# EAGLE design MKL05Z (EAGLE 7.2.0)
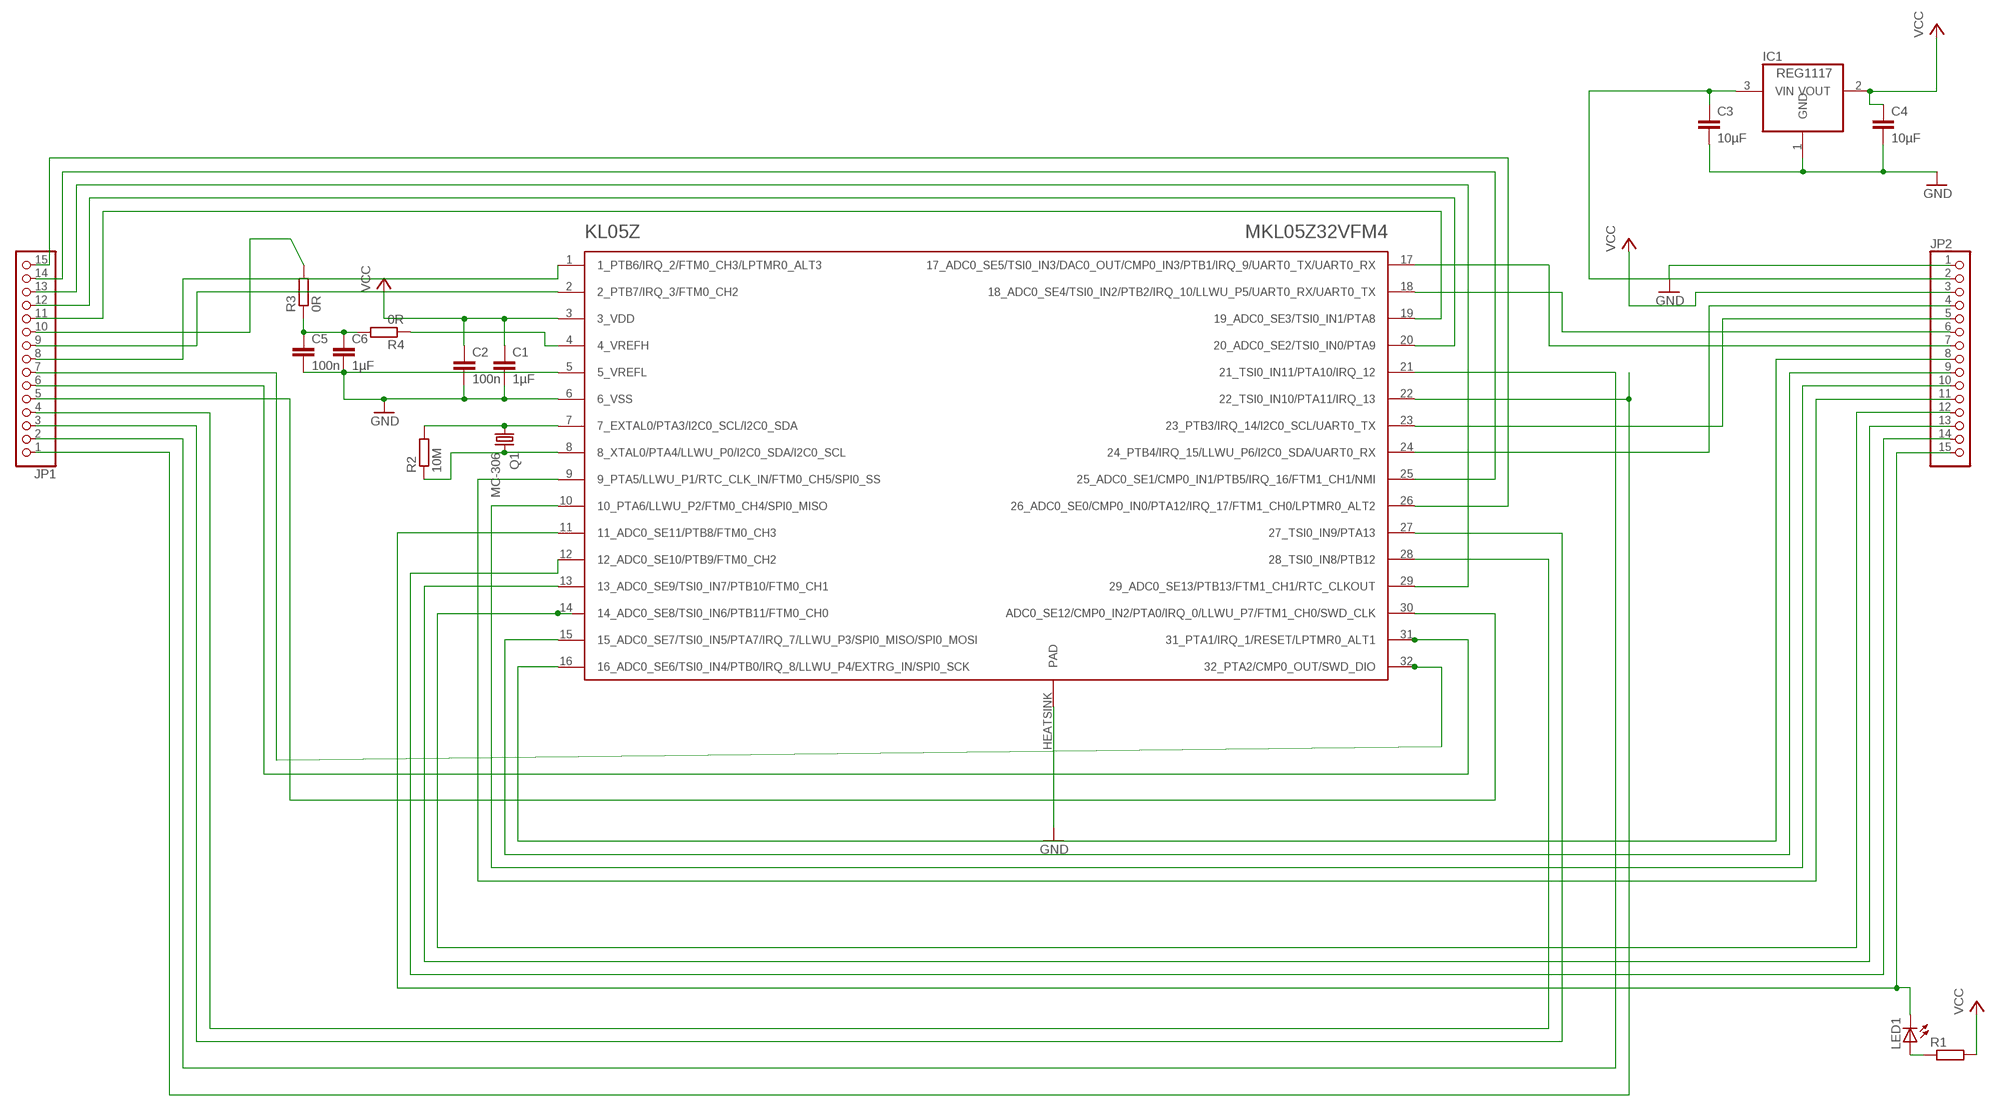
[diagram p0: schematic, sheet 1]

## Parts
C1  1µF  C-EUC0603  [C0603]
C2  100n  C-EUC0603  [C0603]
C3  10µF  C-EUC0805  [C0805]
C4  10µF  C-EUC0805  [C0805]
C5  100n  C-EUC0603  [C0603]
C6  1µF  C-EUC0603  [C0603]
IC1  REG1117  [SOT223]
JP1  PINHD-1X15  [1X15]
JP2  PINHD-1X15  [1X15]
KL05Z  MKL05Z32VFM4  MKL15Z128VFM4  [QFN32]
LED1  LEDCHIPLED_0805  [CHIPLED_0805]
Q1  MC-306  [MC-306]
R1  R-EU_R0603  [R0603]
R2  10M  R-EU_R0603  [R0603]
R3  0R  R-EU_R0402  [R0402]
R4  0R  R-EU_R0402  [R0402]

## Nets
GND: C1.2 C2.2 C3.2 C4.2 C5.2 C6.2 IC1.1(GND) JP2.1 KL05Z.5(5_VREFL) KL05Z.6(6_VSS) KL05Z.HEATSINK(PAD)
N$1: JP1.6 KL05Z.31(31_PTA1/IRQ_1/RESET/LPTMR0_ALT1)
N$2: JP1.4 KL05Z.28(28_TSI0_IN8/PTB12)
N$3: JP1.5 KL05Z.30(ADC0_SE12/CMP0_IN2/PTA0/IRQ_0/LLWU_P7/FTM1_CH0/SWD_CLK)
N$4: KL05Z.7(7_EXTAL0/PTA3/I2C0_SCL/I2C0_SDA) Q1.1 R2.2
N$6: C3.1 IC1.3(VIN) JP2.2
N$7: JP2.6 KL05Z.18(18_ADC0_SE4/TSI0_IN2/PTB2/IRQ_10/LLWU_P5/UART0_RX/UART0_TX)
N$8: JP2.7 KL05Z.17(17_ADC0_SE5/TSI0_IN3/DAC0_OUT/CMP0_IN3/PTB1/IRQ_9/UART0_TX/UART0_RX)
N$9: JP2.4 KL05Z.24(24_PTB4/IRQ_15/LLWU_P6/I2C0_SDA/UART0_RX)
N$10: JP2.5 KL05Z.23(23_PTB3/IRQ_14/I2C0_SCL/UART0_TX)
N$11: KL05Z.8(8_XTAL0/PTA4/LLWU_P0/I2C0_SDA/I2C0_SCL) Q1.4 R2.1
N$12: C5.1 C6.1 R3.1 R4.2
N$13: KL05Z.4(4_VREFH) R4.1
N$14: JP2.11 KL05Z.9(9_PTA5/LLWU_P1/RTC_CLK_IN/FTM0_CH5/SPI0_SS)
N$15: JP2.10 KL05Z.10(10_PTA6/LLWU_P2/FTM0_CH4/SPI0_MISO)
N$16: JP2.9 KL05Z.15(15_ADC0_SE7/TSI0_IN5/PTA7/IRQ_7/LLWU_P3/SPI0_MISO/SPI0_MOSI)
N$17: JP2.8 KL05Z.16(16_ADC0_SE6/TSI0_IN4/PTB0/IRQ_8/LLWU_P4/EXTRG_IN/SPI0_SCK)
N$18: JP1.7 KL05Z.32(32_PTA2/CMP0_OUT/SWD_DIO)
N$19: JP1.3 KL05Z.27(27_TSI0_IN9/PTA13)
N$20: JP1.2 KL05Z.21(21_TSI0_IN11/PTA10/IRQ_12)
N$21: JP1.1 KL05Z.22(22_TSI0_IN10/PTA11/IRQ_13)
N$22: JP1.10 R3.2
N$23: JP1.11 KL05Z.19(19_ADC0_SE3/TSI0_IN1/PTA8)
N$24: JP1.12 KL05Z.20(20_ADC0_SE2/TSI0_IN0/PTA9)
N$25: JP1.13 KL05Z.29(29_ADC0_SE13/PTB13/FTM1_CH1/RTC_CLKOUT)
N$26: JP1.15 KL05Z.26(26_ADC0_SE0/CMP0_IN0/PTA12/IRQ_17/FTM1_CH0/LPTMR0_ALT2)
N$27: JP1.14 KL05Z.25(25_ADC0_SE1/CMP0_IN1/PTB5/IRQ_16/FTM1_CH1/NMI)
N$28: LED1.A R1.1
N$29: JP1.9 KL05Z.2(2_PTB7/IRQ_3/FTM0_CH2)
N$30: JP2.12 KL05Z.14(14_ADC0_SE8/TSI0_IN6/PTB11/FTM0_CH0)
N$31: JP1.8 KL05Z.1(1_PTB6/IRQ_2/FTM0_CH3/LPTMR0_ALT3)
N$32: JP2.13 KL05Z.13(13_ADC0_SE9/TSI0_IN7/PTB10/FTM0_CH1)
N$33: JP2.14 KL05Z.12(12_ADC0_SE10/PTB9/FTM0_CH2)
N$34: JP2.15 KL05Z.11(11_ADC0_SE11/PTB8/FTM0_CH3) LED1.C
VCC: C1.1 C2.1 C4.1 IC1.2(VOUT) JP2.3 KL05Z.3(3_VDD) R1.2

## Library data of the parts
C1-C6 = rcl:C-EU: CAPACITOR, European symbol
IC1 = burr-brown:REG1117: 800mA and 1A Low Dropout (LDO) Positive Regulator 1.8V, 2.5V, 2.85V, 3.3V, 5V, and Adj; MPN: REG1117; OC_FARNELL: 1097566; OC_NEWARK: 14P6981
JP1 JP2 = pinhead:PINHD-1X15: PIN HEADER
KL05Z = kl05z32vfm4:MKL15Z128VFM4
LED1 = led:LED: LED
Q1 = crystal:MC-306: kHz RANGE CRYSTAL UNIT SMD; MPN: MC-306 60.0KHZ 100PPM ,12.5PF; OC_FARNELL: 1278040; OC_NEWARK: 31M5576
R1-R4 = rcl:R-EU_: RESISTOR, European symbol

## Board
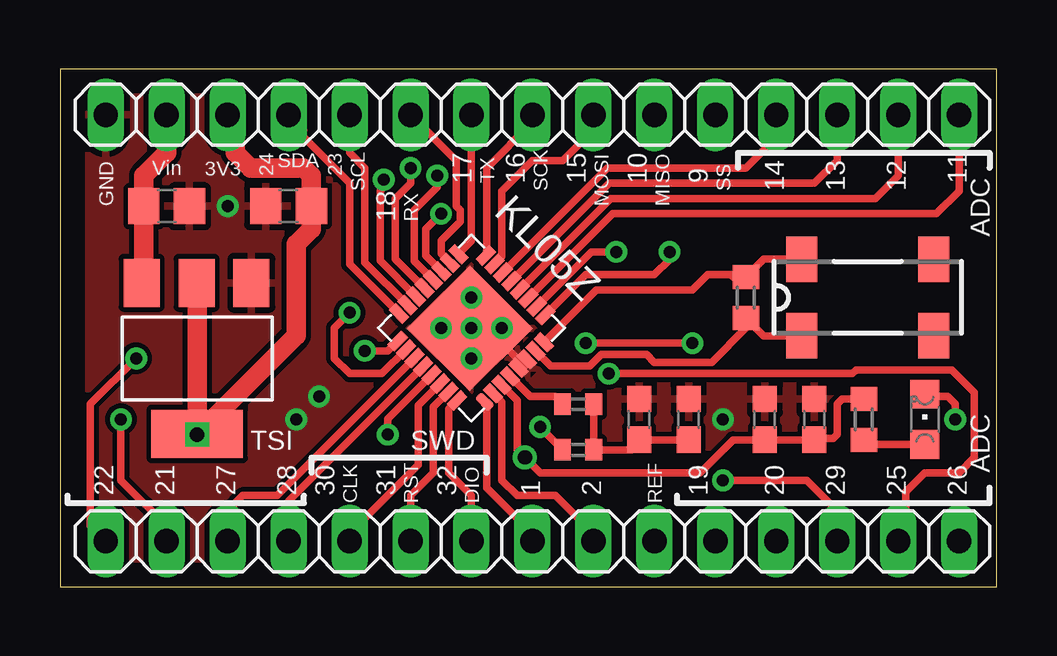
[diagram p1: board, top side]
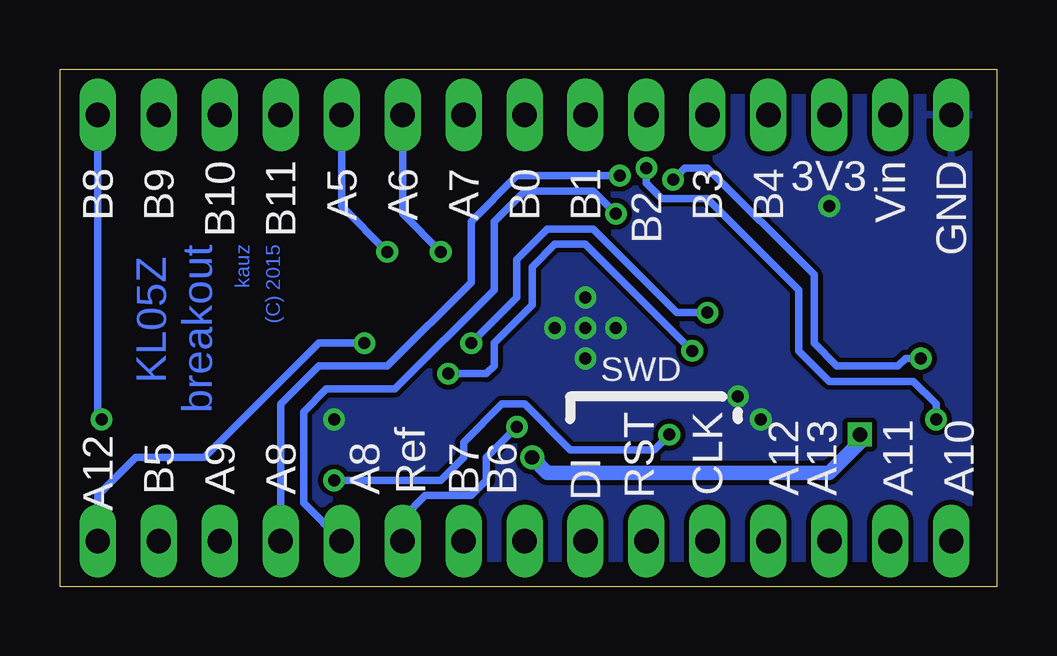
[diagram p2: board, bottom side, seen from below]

Size 39.04 x 21.58 mm. Coordinates in mm from the lower left corner, seen from the top.
Outline: 0,0 39.04,0 39.04,21.58 0,21.58 0,0
Copper layers (1*16): Top 0.035mm / dielectric 1.5mm / Bottom 0.035mm
Design rules "default *": minimum track width 10mil, minimum drill 24mil, track to track 8mil, track to pad 8mil, pad to pad 8mil, via to via 8mil, smd to smd 8mil, copper to edge 40mil, drill to drill 8mil, minimum pad ring 10mil, minimum via ring 8mil, stop-mask expansion 4mil, vias tented up to drill 0.50038125mm, thermal gap 10mil

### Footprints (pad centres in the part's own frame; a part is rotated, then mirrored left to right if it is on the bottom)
C0603 = smd 1.1 x 1: 1 -0.85,0; 2 0.85,0
C0805 = smd 1.3 x 1.5: 1 -0.95,0; 2 0.95,0
SOT223 = smd 1.499 x 2.007: 1 -2.261,-3.15; 2 0.025,-3.15; 3 2.311,-3.15 | smd 3.81 x 2.007: 4 0,3.15
1X15 = drill 1.016 long: 1 -17.78,0; 2 -15.24,0; 3 -12.7,0; 4 -10.16,0; 5 -7.62,0; 6 -5.08,0; 7 -2.54,0; 8 0,0; 9 2.54,0; 10 5.08,0; 11 7.62,0; 12 10.16,0; 13 12.7,0; 14 15.24,0; 15 17.78,0
QFN32 = smd 0.813 x 0.406: 1 -2.56,1.79; 2 -2.56,1.29; 3 -2.56,0.79; 4 -2.56,0.29; 5 -2.56,-0.21; 6 -2.56,-0.71; 7 -2.56,-1.21; 8 -2.56,-1.71; 17 2.56,-1.79; 18 2.56,-1.29; 19 2.56,-0.79; 20 2.56,-0.29; 21 2.56,0.21; 22 2.56,0.71; 23 2.56,1.21; 24 2.56,1.71 | smd 0.406 x 0.813: 9 -1.79,-2.56; 10 -1.29,-2.56; 11 -0.79,-2.56; 12 -0.29,-2.56; 13 0.21,-2.56; 14 0.71,-2.56; 15 1.21,-2.56; 16 1.71,-2.56; 25 1.79,2.56; 26 1.29,2.56; 27 0.79,2.56; 28 0.29,2.56; 29 -0.21,2.56; 30 -0.71,2.56; 31 -1.21,2.56; 32 -1.71,2.56 | smd 3.7 x 3.7: HEATSINK 0.04,0.06
CHIPLED_0805 = smd 1.2 x 1.2: A 0,-1.05; C 0,1.05
MC-306 = smd 1.3 x 1.9: 1 -2.75,-1.6; 2 2.75,-1.6; 3 2.75,1.6; 4 -2.75,1.6
R0603 = smd 1 x 1.1: 1 -0.85,0; 2 0.85,0
R0402 = smd 0.7 x 0.9: 1 -0.65,0; 2 0.65,0

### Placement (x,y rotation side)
C1  29.37,6.99 90 top
C2  31.43,6.99 90 top
C3  4.45,15.88 0 top
C4  9.53,15.88 180 top
C5  26.19,6.99 90 top
C6  24.13,6.99 90 top
IC1  5.71,9.53 180 top
JP1  19.68,1.91 0 top
JP2  19.68,19.68 0 top
KL05Z  17.14,10.79 135 top
LED1  36.04,6.99 0 top
Q1  33.66,12.06 0 top
R1  33.5,6.99 90 top
R2  28.57,12.06 270 top
R3  21.59,5.71 180 top
R4  21.59,7.62 0 top

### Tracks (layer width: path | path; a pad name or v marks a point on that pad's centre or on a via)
GND  (via drill 0.5)
  Top 0.305: KL05Z.6 19.37,9.4 19.37,9.21 18.41,10.16 v18.41,10.79 | v17.14,10.79 17.13,10.78 KL05Z.HEATSINK
  other vias: 9.84,6.99 10.79,7.94 15.88,10.79 17.14,12.06 17.14,9.53 6.99,15.88 27.62,6.99
  pour Top: -1.27,-0.64 -1.27,22.86 40.64,22.86 40.64,-1.27 -1.27,-1.27
  pour Bottom: -0.64,-0.64 -0.64,22.22 40.01,22.22 40.01,0 40.01,-0.64
N$1
  Top 0.305: KL05Z.31 15.56,7.5 15.56,4.76 14.61,3.81 JP1.6
N$2
  Top 0.305: KL05Z.28 9.53,3.58 JP1.4
N$3
  Top 0.305: KL05Z.30 14.92,7.57 14.92,5.08 12.06,2.22 JP1.5
N$4
  Top 0.305: KL05Z.7 20.44,9.21 22.07,9.21 22.54,9.68 24.45,9.68 24.76,9.37 27.15,9.37 28.57,10.79 R2.2 29.32,10.46 Q1.1
N$6
  Top 0.813: IC1.3 3.5,12.77 C3.1 3.49,17.14 4.45,18.1 JP2.2
N$7
  Top 0.305: KL05Z.18 15.88,13.89 15.88,14.45 16.67,15.24 16.67,15.72 16.51,15.88 16.51,17.78 JP2.6
N$8
  Top 0.305: KL05Z.17 17.14,14.42 JP2.7
N$9
  Top 0.305: 10.16,19.05 JP2.4 9.53,19.37 12.06,16.83 12.06,13.46 KL05Z.24
N$10
  Top 0.305: KL05Z.23 12.7,13.53 12.7,17.46 12.06,18.1 JP2.5
N$11
  Top 0.305: KL05Z.8 22.35,12.38 26.35,12.38 26.99,13.02 27.94,13.02 28.04,12.92 R2.1 29.32,13.67 Q1.4
N$12
  Top 0.305: R4.2 R3.1 23.81,5.71 24.13,6.03 C6.1 C5.1
N$13
  Top 0.305: KL05Z.4 19.59,7.94 20.64,7.94 R4.1
N$14  (via drill 0.5)
  Top 0.305: KL05Z.9 21.9,13.02 24.76,13.02 25.4,13.65 v25.4,13.97
  Bottom 0.305: v25.4,13.97 27.3,15.88 JP2.11
N$15  (via drill 0.5)
  Top 0.305: KL05Z.10 22.14,13.97 v23.18,13.97
  Bottom 0.305: v23.18,13.97 24.76,15.56 JP2.10
N$16
  Top 0.305: KL05Z.15 18.41,13.78 18.41,16.51 19.68,17.78 20.95,17.78 22.22,19.05 JP2.9
N$17
  Top 0.305: KL05Z.16 17.78,13.85 17.78,17.46 19.68,19.37 JP2.8
N$18
  Top 0.305: KL05Z.32 16.19,7.42 16.19,4.76 17.14,3.81 JP1.7
N$19
  Top 0.305: KL05Z.27 9.04,3.81 7.62,3.81 6.99,3.17 JP1.3 6.99,1.27
N$20  (via drill 0.5)
  Top 0.305: KL05Z.21 13.97,13.67 13.97,16.19 14.61,16.83 v14.61,17.46 | v2.54,6.99 2.54,4.45 4.45,2.54 JP1.2
  Bottom 0.305: v14.61,17.46 14.61,16.83 13.97,16.19 12.06,16.19 8.26,12.38 8.26,9.84 6.99,8.57 3.49,8.57 2.54,7.62 v2.54,6.99
N$21  (via drill 0.5)
  Top 0.305: KL05Z.22 13.34,13.6 13.34,16.51 13.49,16.67 v13.49,16.99 | JP1.1 1.27,2.54 1.27,7.62 v3.17,9.53
  Bottom 0.305: v13.49,16.99 13.02,17.46 12.06,17.46 7.62,13.02 7.62,10.16 6.67,9.21 4.13,9.21 3.81,9.53 v3.17,9.53
N$22  (via drill 0.5)
  Top 0.305: R3.2 20,6.65 v20,6.67
  Bottom 0.305: v20,6.67 21.27,5.4 21.27,4.45 21.91,3.81 23.81,3.81 24.76,2.86 JP1.10
N$23  (via drill 0.5)
  Top 0.305: KL05Z.19 15.24,13.82 15.24,14.92 v15.88,15.56
  Bottom 0.305: v15.88,15.56 16.83,16.51 19.68,16.51 20.95,15.24 20.95,12.38 25.08,8.26 27.94,8.26 28.89,7.3 28.89,3.49 JP1.11
N$24  (via drill 0.5)
  Top 0.305: KL05Z.20 14.76,13.59 14.76,15.72 15.72,16.67 v15.72,17.14
  Bottom 0.305: v15.72,17.14 20,17.14 21.91,15.24 21.91,12.7 25.4,9.21 28.26,9.21 29.84,7.62 JP1.12
N$25  (via drill 0.5)
  Top 0.305: KL05Z.29 13.65,7.01 v13.65,6.35 | v27.62,4.45 31.11,4.45 32.39,3.17 JP1.13
  Bottom 0.305: v13.65,6.35 14.29,5.71 17.78,5.71 19.68,7.62 20.64,7.62 22.22,6.03 22.22,5.4 23.18,4.45 v27.62,4.45
N$26  (via drill 0.5)
  Top 0.305: v26.35,10.16 v21.91,10.16 | v12.06,11.43 11.43,10.79 11.43,9.53 12.06,8.89 13.42,8.89 KL05Z.26
  Bottom 0.305: JP1.15 37.47,3.81 35.88,5.4 33.02,5.4 28.26,10.16 v26.35,10.16 | v21.91,10.16 20,12.06 20,13.65 18.73,14.92 16.83,14.92 13.34,11.43 v12.06,11.43
N$27  (via drill 0.5)
  Top 0.305: KL05Z.25 13.66,9.84 v12.7,9.84 | v22.86,8.89 33.02,8.89 33.18,9.05 37.15,9.05 38.1,8.1 38.1,5.4 37.47,4.76 36.04,4.76 35.24,3.97 35.24,2.54 34.93,2.22 JP1.14
  Bottom 0.305: v12.7,9.84 17.14,14.29 18.41,14.29 19.37,13.34 19.37,11.75 20.95,10.16 20.95,9.21 21.27,8.89 v22.86,8.89
N$28
  Top 0.305: R1.1 33.7,5.94 LED1.A
N$29
  Top 0.305: KL05Z.2 18.41,7.7 18.41,4.45 19.05,3.81 20.64,3.81 22.22,2.22 JP1.9
N$30
  Top 0.305: KL05Z.14 22.81,17.46 28.57,17.46 29.84,18.73 JP2.12
N$31
  Top 0.305: KL05Z.1 17.78,7.63 17.78,4.13 19.68,2.22 JP1.8
N$32
  Top 0.305: KL05Z.13 22.88,16.83 31.43,16.83 32.39,17.78 JP2.13
N$33
  Top 0.305: KL05Z.12 22.95,16.19 33.97,16.19 34.93,17.14 JP2.14
N$34  (via drill 0.5)
  Top 0.305: KL05Z.11 23.02,15.56 36.51,15.56 37.47,16.51 JP2.15 | LED1.C 36.13,7.94 36.99,7.94 37.31,7.62 v37.31,6.99
  Bottom 0.305: v37.31,6.99 37.47,7.14 JP2.15
VCC  (via drill 0.6)
  Top 0.305: KL05Z.3 19.05,7.77 19.05,5.71 v19.37,5.4 20,4.76 26.67,4.76 28.04,6.13 C1.1 C2.1 31.49,6.19 32.23,6.19 32.39,6.35 32.39,7.62 32.6,7.84 R1.2
  Top 0.813: IC1.2 5.71,12.65 v5.71,6.35 9.84,10.48 9.84,14.29 10.47,14.92 C4.1 10.47,17.15 10.16,17.46 7.94,17.46 7.3,18.1 7.3,19.37 JP2.3
  Bottom 0.61: v19.37,5.4 18.73,4.76 6.99,4.76 5.71,6.03 v5.71,6.35

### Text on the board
Bottom: (C) 2015 | kauz | KL05Z / breakout
tPlace: SDA | Vin | 3V3 | 24 | 23 | GND | SCL | 17 | TX | 16 | SCK | 15 | MOSI | 10 | MISO | 9 | SS | 14 | 13 | 12 | 11 | 18 | RX | ADC | TSI | SWD | ADC | 22 | 21 | 27 | 28 | 30 | CLK | 31 | RST | 32 | DIO | 1 | 2 | REF | 19 | 20 | 29 | 25 | 26
bPlace: GND | Vin | 3V3 | B4 | B3 | B1 | B0 | A7 | A6 | A5 | B11 | B10 | B9 | B8 | B8 | B2 | SWD | A10 | A11 | A13 | A12 | CLK | RST | B6 | B7 | Ref | A8 | A8 | A9 | B5 | A12 | DI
